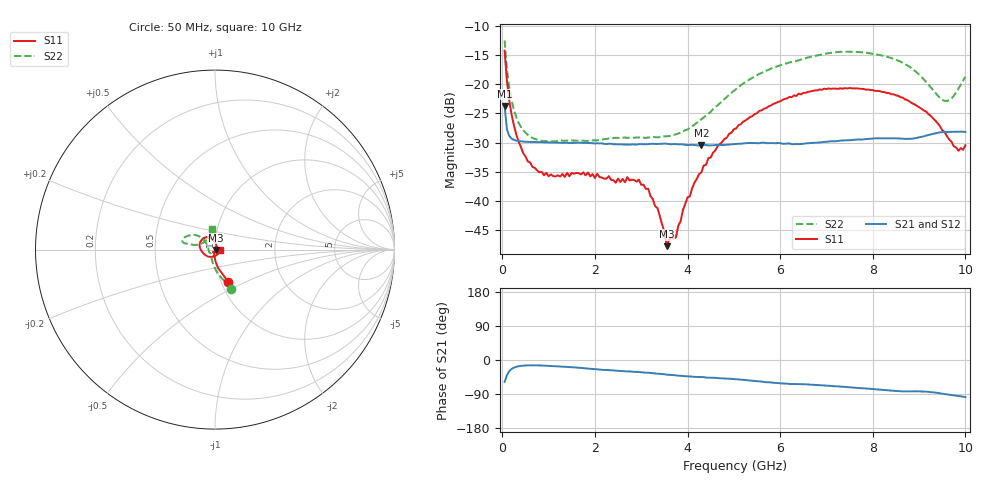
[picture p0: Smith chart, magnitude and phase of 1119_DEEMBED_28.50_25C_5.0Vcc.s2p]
!Hittite Microwave Corp.
!Digital Attenuator/PhaseShifter Rev 1.4.0
!Filename: C:\DATA\DATA\1119_DEEMBED_28.50_25C_5.0Vcc.s2p
!VNA ID: Agilent Technologies,N5224A,MY51441122,A.10.45.03
!Device type:
!2 Port Calibration.
!Temp(C): 25
!Lot Number:
!Serial Number:
!Operator:
!Misc:
!Attenuator:  28.500
# GHZ S DB R 50.0
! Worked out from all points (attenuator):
!   200 points, 50 MHz to 10 GHz, reference 50 ohm
!   highest |S21| = -23.74 dB at 50 MHz (marker M1); lowest = -30.5 dB at 4.3 GHz (marker M2)
!   lowest |S11| = -47.7 dB at 3.55 GHz (marker M3), VSWR 1.01, Z = 50.3 - j0.262 ohm
!   |S11| at or under -10 dB: start of sweep to end of sweep
!   |S22| runs from -29.8 to -12.6 dB; largest |S21 - S12| = 0.00012
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0.05  -14.28 -67.7  -23.74 -57.6  -23.73 -57.6  -12.55 -67.5
0.1  -19.52 -80.0  -27.74 -39.9  -27.74 -39.9  -17.51 -84.0
0.2  -25.18 -89.7  -29.31 -23.7  -29.31 -23.7  -22.78 -100.6
0.35  -29.76 -96.8  -29.73 -16.4  -29.73 -16.5  -26.57 -114.6
0.55  -33.22 -105.2  -29.87 -14.1  -29.86 -14.2  -28.66 -126.4
1  -35.76 -115.5  -29.97 -15.4  -29.97 -15.4  -29.73 -137.3
1.75  -35.07 -120.7  -30.05 -21.6  -30.04 -21.7  -29.67 -140.8
2.95  -36.31 -94.9  -30.26 -31.7  -30.27 -31.9  -29.13 -160.2
3.15  -37.87 -86.4  -30.25 -33.6  -30.26 -33.6  -29.13 -166.2
3.4  -42.50 -77.9  -30.21 -36.4  -30.22 -36.4  -29.05 -173.8
3.55  -47.69 -39.2  -30.19 -38.7  -30.21 -38.8  -28.92 -179.2
3.75  -46.18 25.9  -30.26 -40.6  -30.26 -40.6  -28.58 173.0
4  -39.35 48.0  -30.40 -43.0  -30.40 -43.1  -27.76 161.8
4.3  -35.06 65.3  -30.49 -44.9  -30.51 -45.1  -25.99 150.4
5.05  -27.58 89.4  -30.23 -50.8  -30.25 -50.8  -20.83 138.6
5.85  -23.40 111.5  -30.08 -60.1  -30.08 -60.1  -17.19 143.9
6.7  -21.18 130.8  -30.04 -65.3  -30.05 -65.3  -15.26 153.8
8.35  -21.54 174.4  -29.28 -80.3  -29.28 -80.3  -15.44 168.1
9.15  -24.69 -142.4  -28.81 -83.5  -28.83 -83.6  -19.61 165.4
9.55  -28.23 -98.3  -28.19 -89.9  -28.21 -89.9  -22.86 138.1
9.85  -31.40 -38.7  -28.14 -94.9  -28.14 -94.9  -20.76 105.8
10  -30.45 -4.0  -28.18 -97.7  -28.19 -97.7  -18.74 98.2
